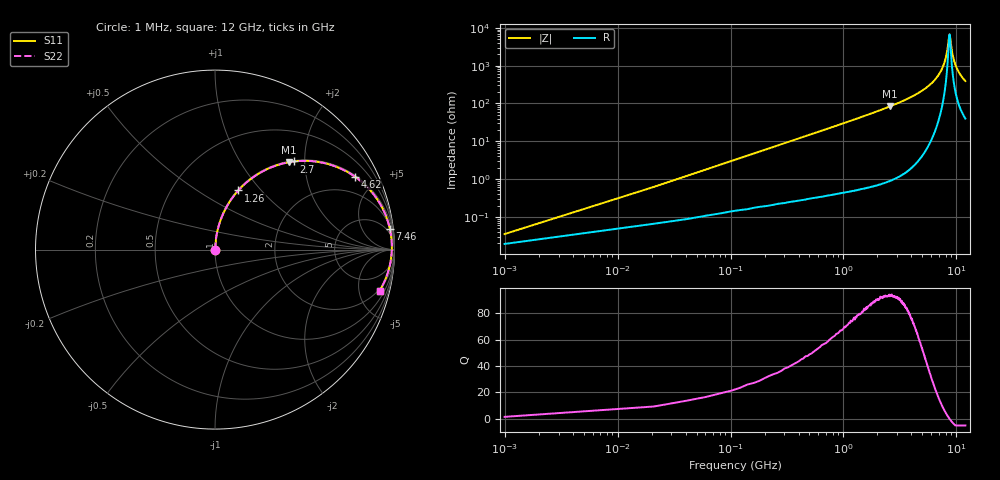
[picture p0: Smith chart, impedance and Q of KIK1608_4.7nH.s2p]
!version-2
!date-01.2022
!Series
# MHz S RI R 50
!Freq ReS11 ImS11 ReS21 ImS21 ReS12 ImS12 ReS22 ImS22
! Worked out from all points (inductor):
!   601 points, 1 MHz to 12 GHz, reference 50 ohm
!   read as one part in series: L = 4.7 nH near 61 MHz
!   highest Q = 93.2 at 2.58 GHz (marker M1), where L = 5.16 nH
!   self-resonance near 8.692 GHz
!   S11 on the Smith chart (normalised r, x): 1 MHz: 1.00, +0.00; 1.26 GHz: 1.01, +0.76; 2.7 GHz: 1.02, +1.77; 4.62 GHz: 1.06, +3.80; 7.46 GHz: 3, +17; 12 GHz: 1.79, -7.76
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1  0.000187 0.000295  0.9998 -0.000295  0.9998 -0.000295  0.000187 0.000295
81  0.00181 0.0238  0.9982 -0.0238  0.9982 -0.0238  0.00181 0.0238
141  0.00334 0.0414  0.9967 -0.0414  0.9967 -0.0414  0.00334 0.0414
241  0.00712 0.0706  0.9929 -0.0706  0.9929 -0.0706  0.00712 0.0706
401  0.0165 0.1164  0.9835 -0.1164  0.9835 -0.1164  0.0165 0.1164
621  0.0359 0.1771  0.9641 -0.1771  0.9641 -0.1771  0.0359 0.1771
1260  0.1297 0.3294  0.8703 -0.3294  0.8703 -0.3294  0.1297 0.3294
2020  0.2869 0.4468  0.7131 -0.4468  0.7131 -0.4468  0.2869 0.4468
2580  0.4123 0.4869  0.5877 -0.4869  0.5877 -0.4869  0.4123 0.4869
2700  0.4387 0.4909  0.5613 -0.4909  0.5613 -0.4909  0.4387 0.4909
4020  0.6931 0.4546  0.3069 -0.4546  0.3069 -0.4546  0.6931 0.4546
4620  0.7798 0.4063  0.2202 -0.4063  0.2202 -0.4063  0.7798 0.4063
6020  0.9139 0.2647  0.0861 -0.2647  0.0861 -0.2647  0.9139 0.2647
7460  0.9746 0.115  0.0254 -0.115  0.0254 -0.115  0.9746 0.115
8020  0.9831 0.0608  0.0169 -0.0608  0.0169 -0.0608  0.9831 0.0608
8300  0.985 0.0349  0.015 -0.0349  0.015 -0.0349  0.985 0.0349
8600  0.9854 0.00803  0.0146 -0.00803  0.0146 -0.00803  0.9854 0.00803
8700  0.9852 -0.000706  0.0148 0.000706  0.0148 0.000706  0.9852 -0.000706
9280  0.9812 -0.0492  0.0188 0.0492  0.0188 0.0492  0.9812 -0.0492
10020  0.9699 -0.1056  0.0301 0.1056  0.0301 0.1056  0.9699 -0.1056
10860  0.9509 -0.1625  0.0491 0.1625  0.0491 0.1625  0.9509 -0.1625
12000  0.9179 -0.2281  0.0822 0.2281  0.0822 0.2281  0.9179 -0.2281
